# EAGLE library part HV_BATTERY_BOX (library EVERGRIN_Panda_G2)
HV battery box
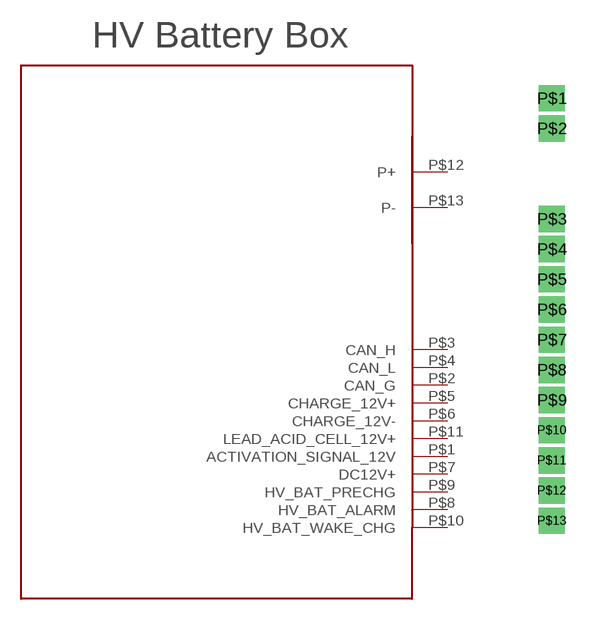
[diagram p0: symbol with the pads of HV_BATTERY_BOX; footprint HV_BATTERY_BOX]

Designator prefix -

## HV_BATTERY_BOX  [HV_BATTERY_BOX]
P$1  ACTIVATION_SIGNAL_12V
P$2  CAN_G
P$3  CAN_H
P$4  CAN_L
P$5  CHARGE_12V+
P$6  CHARGE_12V-
P$7  DC12V+
P$8  HV_BAT_ALARM
P$9  HV_BAT_PRECHG
P$10  HV_BAT_WAKE_CHG
P$11  LEAD_ACID_CELL_12V+
P$12  P+  pwr
P$13  P-  pwr

## Footprint HV_BATTERY_BOX (pad centres in mm)
drill 0.6 square: P$1 0,17.78; P$2 0,16.51; P$3 0,12.7; P$4 0,11.43; P$5 0,10.16; P$6 0,8.89; P$7 0,7.62; P$8 0,6.35; P$9 0,5.08; P$10 0,3.81; P$11 0,2.54; P$12 0,1.27; P$13 0,0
